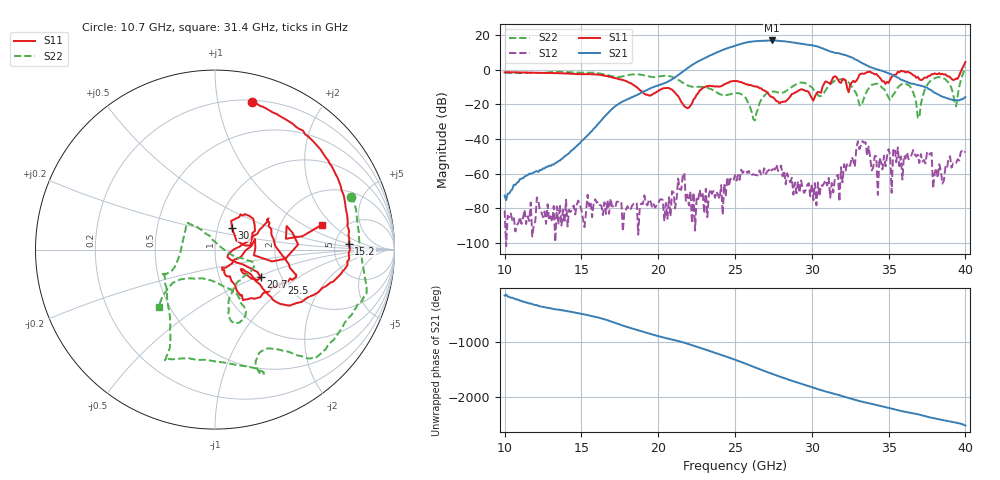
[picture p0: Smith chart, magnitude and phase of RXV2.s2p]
!Keysight Technologies,M9808A,MY58100618,A.14.70.03
!Date: Monday, February 27, 2023 13:25:24
!Correction: S11(Cdelta 2-Port  )
!S21(Cdelta 2-Port  )
!S12(Cdelta 2-Port  )
!S22(Cdelta 2-Port  )
!S2P File: Measurements: S11, S21, S12, S22:
# Hz S  RI  R 50
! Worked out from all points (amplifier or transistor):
!   301 points, 10 GHz to 40 GHz, reference 50 ohm
!   highest |S21| = 16.9 dB at 27.4 GHz (marker M1)
!   |S21| within 3 dB of that: 25.03 GHz to 30.13 GHz (5.104 GHz wide, 18.5 % of centre)
!   unconditionally stable (mu >= 1): start of sweep to 39.73 GHz
!   at 15 GHz: K = 86862.25, MAG = -32.6 dB, |S12| = -80.9 dB
!   at 25 GHz: K = 83.08, MAG = 15.2 dB, |S12| = -60.9 dB
!   at 40 GHz: K = 612.48, MSG = 15.7 dB, |S12| = -47.2 dB
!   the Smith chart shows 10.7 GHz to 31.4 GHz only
!   S11 on the Smith chart (normalised r, x): 10.7 GHz: 0.21, +1.26; 15.2 GHz: 6.75, +0.92; 20.7 GHz: 1.58, -0.53; 25.5 GHz: 1.94, -0.87; 30 GHz: 1.17, +0.29; 31.4 GHz: 3.42, +1.50
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1e10  0.0862 0.844  -0.000204 -0.000117  -7.55e-05 -4.23e-05  0.6918 0.4549
1.07e10  0.2068 0.8245  -0.000397 0.000256  -6.49e-06 -2.06e-05  0.7554 0.2934
1.5e10  0.7438 0.0814  -0.00486 -0.00718  4.56e-05 -7.84e-05  0.6598 -0.5043
1.52e10  0.7455 0.0303  -0.00745 -0.00727  1.86e-05 2.2e-05  0.627 -0.537
2e10  0.1906 -0.1522  -0.3511 -0.0463  9.97e-05 9.48e-05  -0.1788 -0.6059
2.07e10  0.255 -0.1527  -0.3551 0.3103  -0.000167 0.000126  -0.272 -0.6
2.27e10  0.2372 0.0895  1.698 -0.7187  0.000169 -0.000299  -0.2972 -0.1274
2.37e10  0.2982 0.1315  -1.324 -2.706  -0.000148 0.000136  -0.2191 -0.0883
2.44e10  0.3911 -0.054  -4.009 0.2612  -6.66e-05 0.000228  -0.177 0.0577
2.5e10  0.4497 -0.1472  -2.202 4.414  -1.48e-05 0.000904  -0.1608 0.1403
2.55e10  0.374 -0.1844  2.423 5.201  0.000599 0.000869  -0.1247 0.1361
2.63e10  0.1776 -0.2776  6.149 -2.657  0.00091 0.00015  0.0312 0.0149
2.69e10  0.1201 -0.2232  0.2513 -6.94  0.00127 0.000683  0.1665 -0.0538
2.74e10  0.0703 -0.1497  -5.333 -4.575  0.00128 0.000292  0.2173 -0.0944
2.8e10  0.0589 -0.1009  -6.319 2.371  0.00172 8.35e-05  0.1456 -0.1691
2.86e10  0.1701 -0.00484  -1.271 6.185  0.000447 -0.000353  0.0778 -0.2764
2.93e10  0.2129 0.1718  4.368 3.543  0.000624 0.000152  0.1366 -0.4069
3e10  0.0951 0.12  4.68 -2.056  -0.00016 0.000495  0.1396 -0.279
3.14e10  0.5947 0.1379  -2.528 -1.945  0.00013 0.000255  -0.3135 -0.3214
3.27e10  0.4683 -0.1125  -0.8509 1.993  -0.00176 0.00166  0.000969 -0.2921
3.5e10  0.3673 -0.1996  0.5622 -0.5603  -0.00498 0.00116  0.00646 -0.1586
4e10  0.6377 -1.553  0.1629 -0.0118  0.00174 0.00402  0.6057 -1.055
